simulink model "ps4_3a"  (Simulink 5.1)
settings: Solver=ode45  StartTime=0.0  StopTime=10.0  RelTol=1e-3
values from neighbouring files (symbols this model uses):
  d = 0.0001    [ps4_3.m]
  s = tf('s')    [ps7_3_2.m]    (also in ps4_2.m; ps7_1_2.m; ps4_3.m; ps2_3.m)
libraries: cstblocks x6

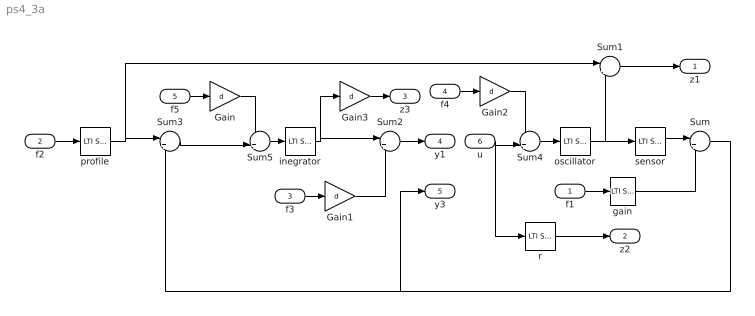
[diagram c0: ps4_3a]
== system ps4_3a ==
  f1 : Inport
  f2 : Inport  Port=2
  f3 : Inport  Port=3
  f4 : Inport  Port=4
  f5 : Inport  Port=5
  u : Inport  Port=6
  Gain{,1..3} (4 alike) : Gain  Gain=d
  Sum : Sum  Inputs=|++
  Sum1 : Sum  Inputs=|+-
  Sum2 : Sum  Inputs=|++
  Sum3 : Sum  Inputs=|+-
  Sum4 : Sum  Inputs=++|
  Sum5 : Sum  Inputs=++|
  gain : cstblocks/LTI System  sys=0.1  IC=[]
  inegrator : cstblocks/LTI System  sys=1/s  IC=[]
  oscillator : cstblocks/LTI System  sys=P0  IC=[]
  profile : cstblocks/LTI System  sys=P2  IC=[]
  r : cstblocks/LTI System  sys=r  IC=[]
  sensor : cstblocks/LTI System  sys=P1  IC=[]
  z1 : Outport
  z2 : Outport  Port=2
  z3 : Outport  Port=3
  y1 : Outport  Port=4
  y3 : Outport  Port=5
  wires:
  oscillator/1 -> sensor/1, Sum1/2
  sensor/1 -> Sum/1
  gain/1 -> Sum/2
  f1/1 -> gain/1
  f2/1 -> profile/1
  f3/1 -> Gain1/1
  profile/1 -> Sum1/1, Sum3/1
  inegrator/1 -> Sum2/1, Gain3/1
  Gain1/1 -> Sum2/2
  r/1 -> z2/1
  Sum1/1 -> z1/1
  Sum2/1 -> y1/1
  Sum/1 -> Sum3/2, y3/1
  f4/1 -> Gain2/1
  Gain2/1 -> Sum4/1
  Sum4/1 -> oscillator/1
  Sum5/1 -> inegrator/1
  Sum3/1 -> Sum5/2
  Gain/1 -> Sum5/1
  f5/1 -> Gain/1
  u/1 -> Sum4/2, r/1
  Gain3/1 -> z3/1
